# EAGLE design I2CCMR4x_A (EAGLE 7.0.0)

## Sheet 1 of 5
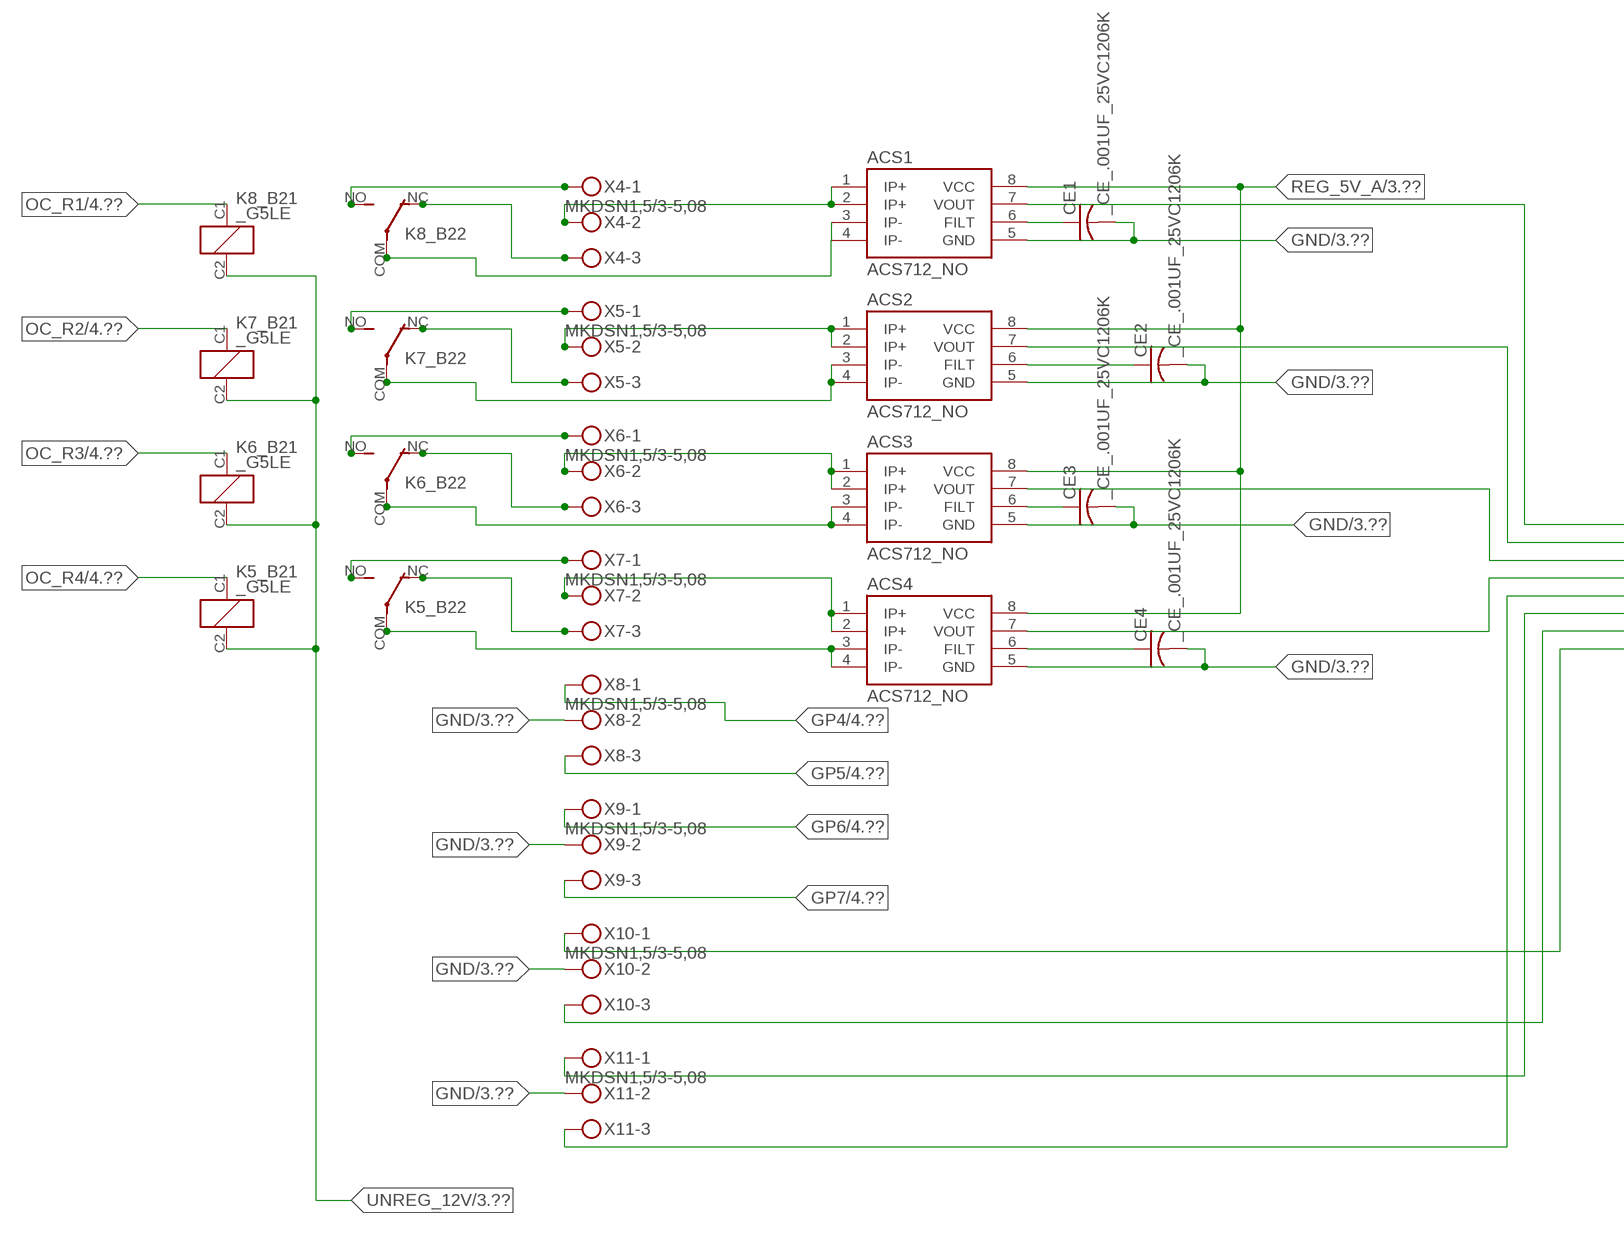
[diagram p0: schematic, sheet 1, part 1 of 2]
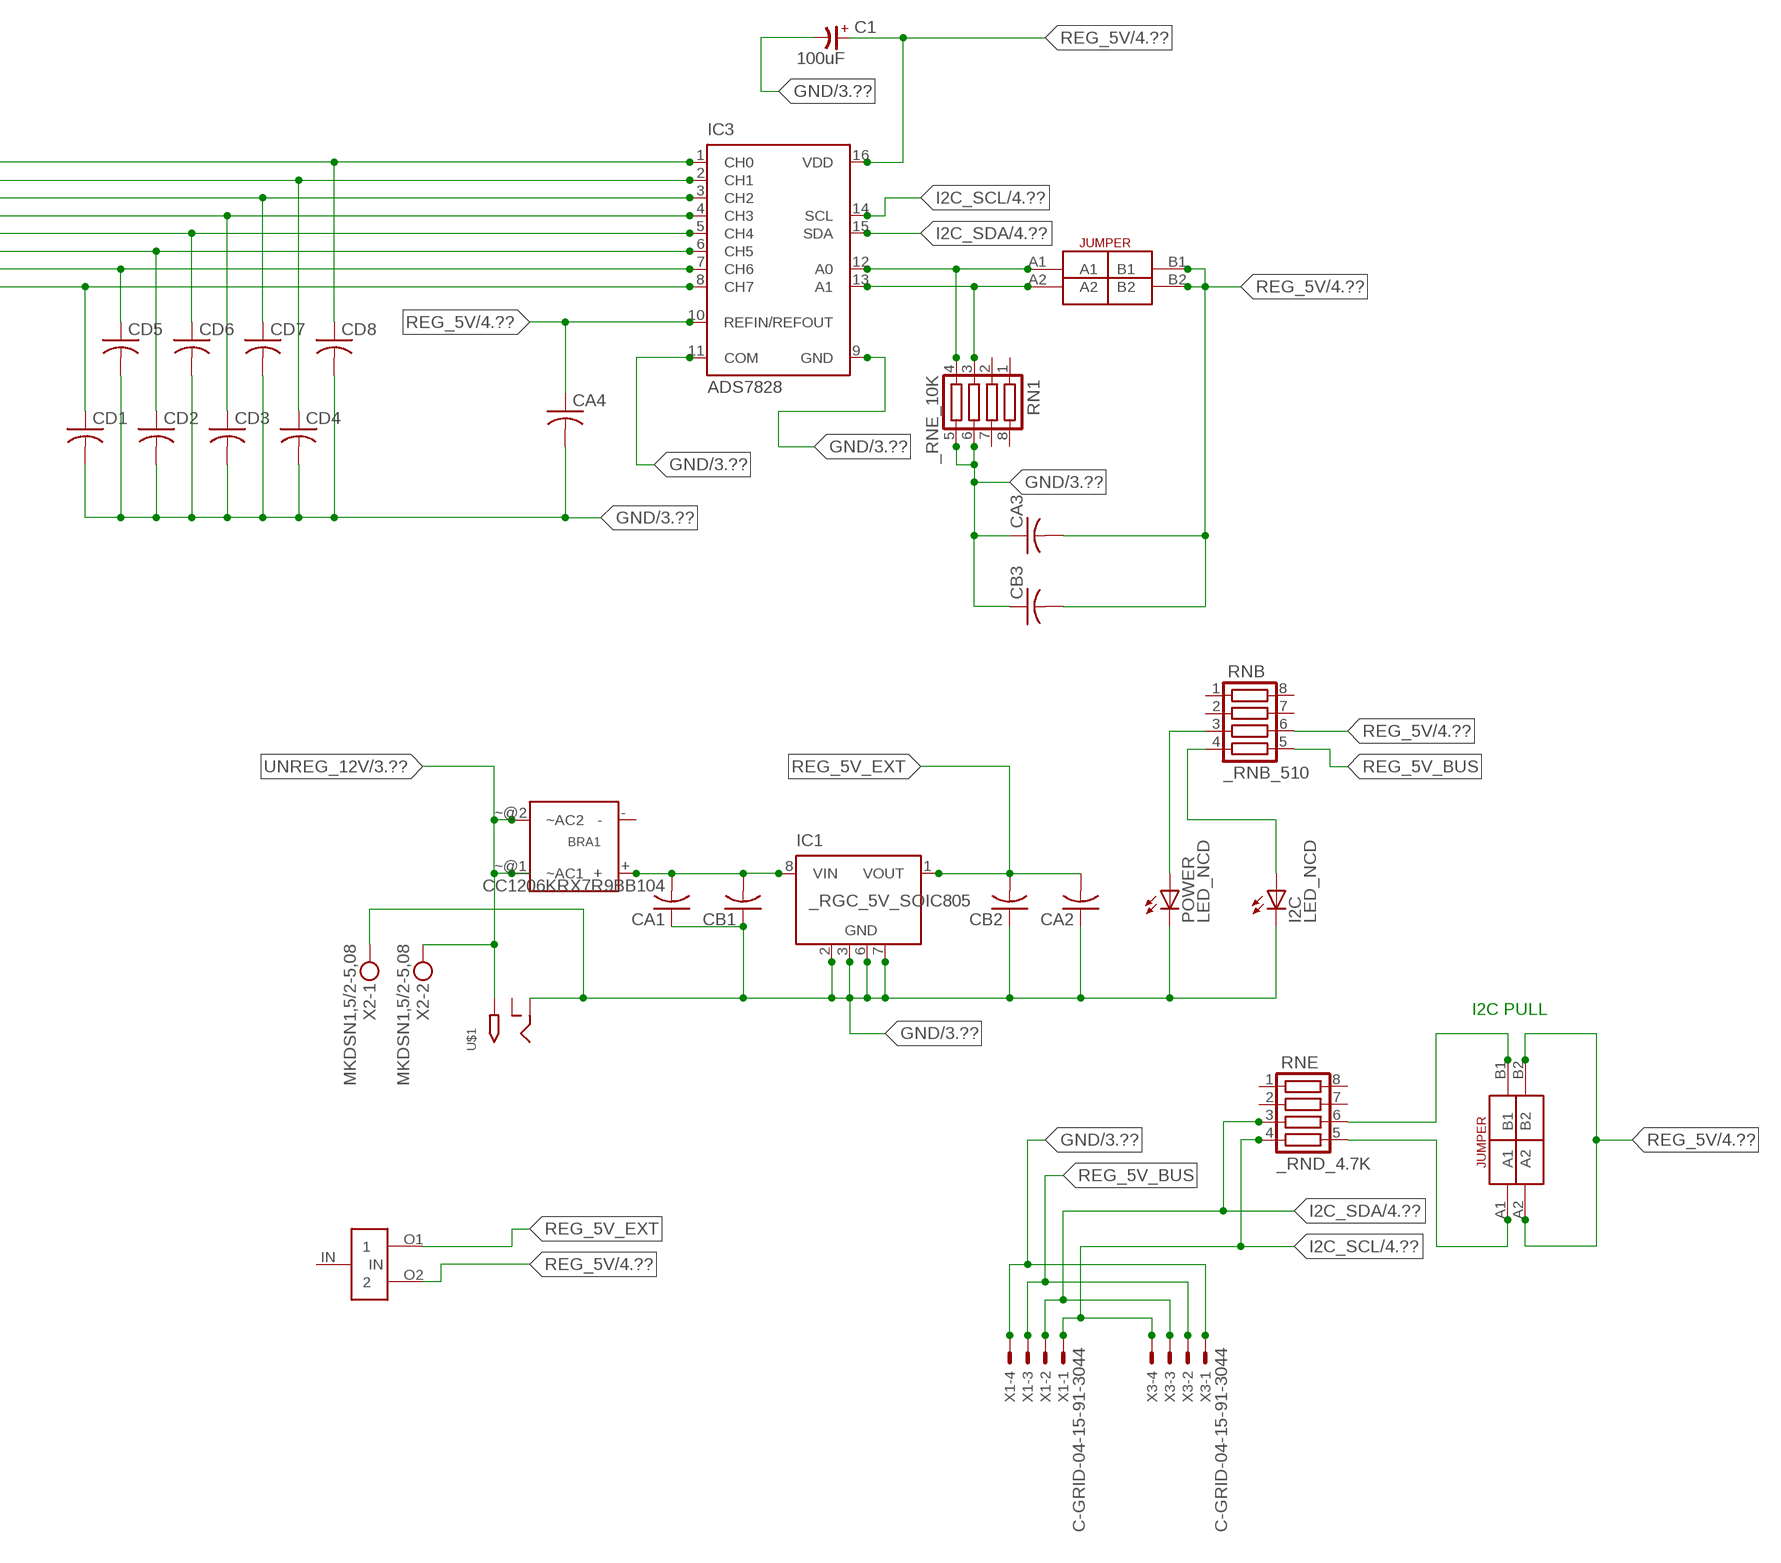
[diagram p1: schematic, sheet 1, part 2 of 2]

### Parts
ACS1  ACS712_NO  [_MA_DUAL_N-FET]
ACS2  ACS712_NO  [_MA_DUAL_N-FET]
ACS3  ACS712_NO  [_MA_DUAL_N-FET]
ACS4  ACS712_NO  [_MA_DUAL_N-FET]
BRA1  MB2S_  [MB2S]
C1  100uF  CP-E-025X060  [E-025X060]
CA1  CC1206KRX7R9BB104  [.1UF]
CA2  CC1206KRX7R9BB104C1206K  [CC1206KRX7R9BB104]
CA3  CC1206KRX7R9BB104C1206K  [CC1206KRX7R9BB104]
CA4  CC1206KRX7R9BB104C1206K  [CC1206KRX7R9BB104]
CB1  TMK316F106ZL-TC1206K  [TMK316F106ZL-T]
CB2  TMK316F106ZL-TC1206K  [TMK316F106ZL-T]
CB3  TMK316F106ZL-TC1206K  [TMK316F106ZL-T]
CD1  _CD_10NF_50VC1206K  [_CD_10NF_50V]
CD2  _CD_10NF_50VC1206K  [_CD_10NF_50V]
CD3  _CD_10NF_50VC1206K  [_CD_10NF_50V]
CD4  _CD_10NF_50VC1206K  [_CD_10NF_50V]
CD5  _CD_10NF_50VC1206K  [_CD_10NF_50V]
CD6  _CD_10NF_50VC1206K  [_CD_10NF_50V]
CD7  _CD_10NF_50VC1206K  [_CD_10NF_50V]
CD8  _CD_10NF_50VC1206K  [_CD_10NF_50V]
CE1  _CE_.001UF_25VC1206K  [CE]
CE2  _CE_.001UF_25VC1206K  [CE]
CE3  _CE_.001UF_25VC1206K  [CE]
CE4  _CE_.001UF_25VC1206K  [CE]
I2C  LED_NCD  [CHIPLED_0603]
IC1  _RGC_5V_SOIC805  [_RGC_5V_SOIC8]
IC3  ADS7828  [TSSOP16-PW]
K5_B2  _G5LE  [G5LE]
K6_B2  _G5LE  [G5LE]
K7_B2  _G5LE  [G5LE]
K8_B2  _G5LE  [G5LE]
POWER  LED_NCD  [CHIPLED_0603]
RN1  _RNE_10K  [RNE]
RNB  _RNB_510  [RNB]
RNE  _RND_4.7K  [RND]
U$1  2.1MMJACK  [PJ-102A]
U$2  LINK_2  [LINK_2]
U$3  JUMPER_2X2  [JUMPER_2X2]
U$4  JUMPER_2X2  [JUMPER_2X2]
X1  C-GRID-04-15-91-3044  [15-91-04]
X2  MKDSN1,5/2-5,08  [MKDSN1,5/2-5,08]
X3  C-GRID-04-15-91-3044  [15-91-04]
X4  MKDSN1,5/3-5,08  [MKDSN1,5/3-5,08]
X5  MKDSN1,5/3-5,08  [MKDSN1,5/3-5,08]
X6  MKDSN1,5/3-5,08  [MKDSN1,5/3-5,08]
X7  MKDSN1,5/3-5,08  [MKDSN1,5/3-5,08]
X8  MKDSN1,5/3-5,08  [MKDSN1,5/3-5,08]
X9  MKDSN1,5/3-5,08  [MKDSN1,5/3-5,08]
X10  MKDSN1,5/3-5,08  [MKDSN1,5/3-5,08]
X11  MKDSN1,5/3-5,08  [MKDSN1,5/3-5,08]

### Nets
GND: ACS1.5(GND) ACS2.5(GND) ACS3.5(GND) ACS4.5(GND) C1.- CA1.1 CA2.1 CA3.1 CA4.2 CB1.1 CB2.1 CB3.1 CD1.2 CD2.2 CD3.2 CD4.2 CD5.2 CD6.2 CD7.2 CD8.2 CE1.2 CE2.2 CE3.2 CE4.2 I2C.C IC1.2(GND) IC1.3(GND) IC1.6(GND) IC1.7(GND) IC3.9(GND) IC3.11(COM) POWER.C RN1.5 RN1.6 U$1.RING X1.4 X2.1 X3.1 X8.2 X9.2 X10.2 X11.2 ; also sheet 3,4
GP4: X8.1 ; also sheet 4
GP5: X8.3 ; also sheet 4
GP6: X9.1 ; also sheet 4
GP7: X9.3 ; also sheet 4
I2C_SCL: IC3.14(SCL) RNE.4 X1.1 X3.4 ; also sheet 4
I2C_SDA: IC3.15(SDA) RNE.3 X1.2 X3.3 ; also sheet 4
N$1: BRA1.+ CA1.2 CB1.2 IC1.8(VIN)
N$2: POWER.A RNB.3
N$3: I2C.A RNB.4
N$4: RNE.5 U$3.A1
N$5: RNE.6 U$3.B1
N$7: ACS1.1(IP+) ACS1.2(IP+) X4.2
N$8: CD5.1 IC3.7(CH6) X10.3
N$9: ACS1.7(VOUT) CD8.1 IC3.1(CH0)
N$10: ACS2.7(VOUT) CD4.1 IC3.2(CH1)
N$11: ACS3.7(VOUT) CD7.1 IC3.3(CH2)
N$12: ACS4.7(VOUT) CD3.1 IC3.4(CH3)
N$13: ACS2.1(IP+) ACS2.2(IP+) X5.2
N$17: IC3.12(A0) RN1.4 U$4.A1
N$18: IC3.13(A1) RN1.3 U$4.A2
N$20: CD2.1 IC3.6(CH5) X11.1
N$21: ACS4.1(IP+) ACS4.2(IP+) X7.2
N$22: ACS4.3(IP-) ACS4.4(IP-) K5_B2.COM(2:COM)
N$24: CD1.1 IC3.8(CH7) X10.1
N$25: CD6.1 IC3.5(CH4) X11.3
N$33: ACS1.6(FILT) CE1.1
N$34: ACS2.6(FILT) CE2.1
N$35: ACS3.6(FILT) CE3.1
N$36: ACS4.6(FILT) CE4.1
N$42: ACS1.3(IP-) ACS1.4(IP-) K8_B2.COM(2:COM)
N$43: K8_B2.NC(2:NC) X4.3
N$44: K8_B2.NO(2:NO) X4.1
N$45: K7_B2.NO(2:NO) X5.1
N$46: K6_B2.NO(2:NO) X6.1
N$137: K7_B2.NC(2:NC) X5.3
N$138: ACS2.3(IP-) ACS2.4(IP-) K7_B2.COM(2:COM)
N$139: K6_B2.NC(2:NC) X6.3
N$140: ACS3.3(IP-) ACS3.4(IP-) K6_B2.COM(2:COM)
N$141: K5_B2.NC(2:NC) X7.3
N$143: K5_B2.NO(2:NO) X7.1
N$166: ACS3.1(IP+) ACS3.2(IP+) X6.2
OC_R1: K8_B2.C1(1:C1) ; also sheet 4
OC_R2: K7_B2.C1(1:C1) ; also sheet 4
OC_R3: K6_B2.C1(1:C1) ; also sheet 4
OC_R4: K5_B2.C1(1:C1) ; also sheet 4
REG_5V: C1.+ CA3.2 CA4.1 CB3.2 IC3.10(REFIN/REFOUT) IC3.16(VDD) RNB.6 U$2.O2 U$3.A2 U$3.B2 U$4.B1 U$4.B2 ; also sheet 4
REG_5V_A: ACS1.8(VCC) ACS2.8(VCC) ACS3.8(VCC) ACS4.8(VCC) ; also sheet 3
REG_5V_BUS: RNB.5 X1.3 X3.2
REG_5V_EXT: CA2.2 CB2.2 IC1.1(VOUT) U$2.O1
UNREG_12V: BRA1.~@1(~AC1) BRA1.~@2(~AC2) K5_B2.C2(1:C2) K6_B2.C2(1:C2) K7_B2.C2(1:C2) K8_B2.C2(1:C2) U$1.TIP X2.2 ; also sheet 3,4
Unconnected: BRA1.- IC1.4(NC) IC1.5(NC) RN1.1 RN1.2 RN1.7 RN1.8 RNB.1 RNB.2 RNB.7 RNB.8 RNE.1 RNE.2 RNE.7 RNE.8 U$1.RING_SW U$2.IN

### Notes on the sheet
- I2C PULL

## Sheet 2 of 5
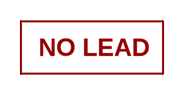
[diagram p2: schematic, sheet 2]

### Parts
U$16  NOPB_LOGO_SYM  [NOPB_LOGO_SYM]

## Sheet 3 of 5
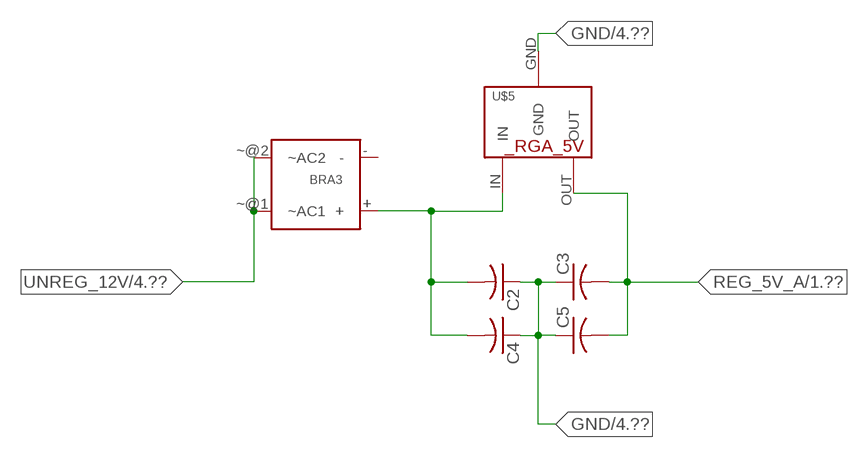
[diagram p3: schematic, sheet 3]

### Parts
BRA3  MB2S_  [MB2S]
C2  _CA_.10UF_50VC1206K  [_CA_.1UF_50V]
C3  _CA_.10UF_50VC1206K  [_CA_.1UF_50V]
C4  _CB_10UF_25VC1206K  [_CB_10UF_25V]
C5  _CB_10UF_25VC1206K  [_CB_10UF_25V]
U$5  _RGA_5V  [_RGA_5V]

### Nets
GND: C2.1 C3.1 C4.1 C5.1 U$5.GND ; also sheet 1,4
N$31: BRA3.+ C2.2 C4.2 U$5.IN
REG_5V_A: C3.2 C5.2 U$5.OUT ; also sheet 1
UNREG_12V: BRA3.~@1(~AC1) BRA3.~@2(~AC2) ; also sheet 1,4
Unconnected: BRA3.-

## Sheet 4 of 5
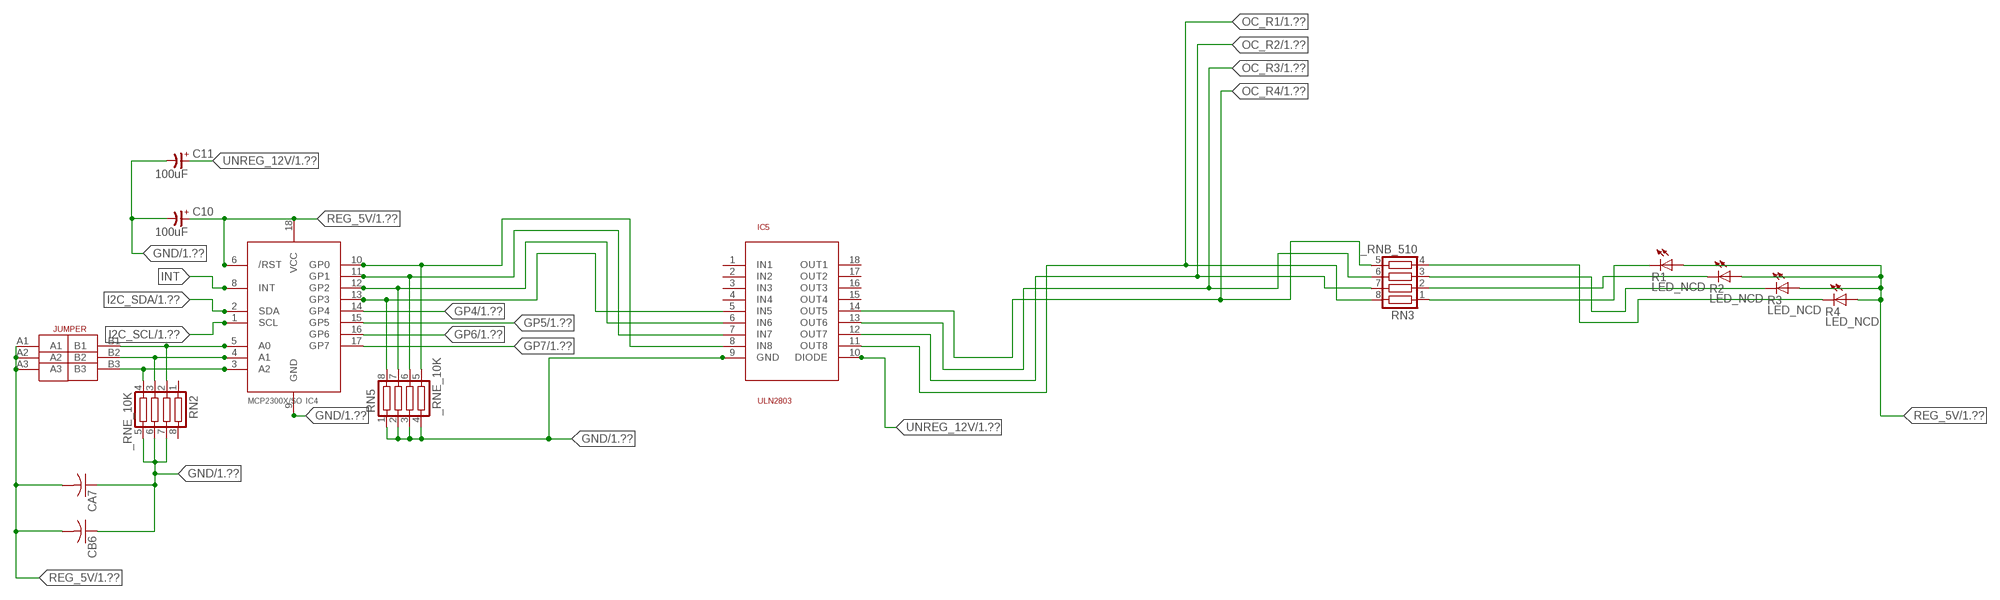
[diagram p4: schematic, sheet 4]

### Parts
C10  100uF  CP-E-025X060  [E-025X060]
C11  100uF  CP-E-025X060  [E-025X060]
CA7  CC1206KRX7R9BB104C1206K  [CC1206KRX7R9BB104]
CB6  TMK316F106ZL-TC1206K  [TMK316F106ZL-T]
IC4  MCP2300X/SO  [SO18W]
IC5  ULN2803  [SO18L]
R1  LED_NCD  [CHIPLED_0603]
R2  LED_NCD  [CHIPLED_0603]
R3  LED_NCD  [CHIPLED_0603]
R4  LED_NCD  [CHIPLED_0603]
RN2  _RNE_10K  [RNE]
RN3  _RNB_510  [RNB]
RN5  _RNE_10K  [RNE]
U$18  JUMPER_3X2  [JUMPER_3X2]

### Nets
GND: C10.- C11.- CA7.1 CB6.1 IC4.9(GND) IC5.9(GND) RN2.5 RN2.6 RN2.7 RN5.1 RN5.2 RN5.3 RN5.4 ; also sheet 1,3
GP4: IC4.14(GP4) ; also sheet 1
GP5: IC4.15(GP5) ; also sheet 1
GP6: IC4.16(GP6) ; also sheet 1
GP7: IC4.17(GP7) ; also sheet 1
I2C_SCL: IC4.1(SCL) ; also sheet 1
I2C_SDA: IC4.2(SDA) ; also sheet 1
INT: IC4.8(INT)
N$47: IC4.5(A0) RN2.2 U$18.B1
N$48: IC4.4(A1) RN2.3 U$18.B2
N$49: IC4.3(A2) RN2.4 U$18.B3
N$50: IC4.12(GP2) IC5.6(IN6) RN5.7
N$51: IC4.11(GP1) IC5.7(IN7) RN5.6
N$52: IC4.10(GP0) IC5.8(IN8) RN5.5
N$53: R1.C RN3.1
N$54: R2.C RN3.2
N$55: R3.C RN3.3
N$56: R4.C RN3.4
N$89: IC4.13(GP3) IC5.5(IN5) RN5.8
OC_R1: IC5.11(OUT8) RN3.8 ; also sheet 1
OC_R2: IC5.12(OUT7) RN3.7 ; also sheet 1
OC_R3: IC5.13(OUT6) RN3.6 ; also sheet 1
OC_R4: IC5.14(OUT5) RN3.5 ; also sheet 1
REG_5V: C10.+ CA7.2 CB6.2 IC4.6(/RST) IC4.18(VCC) R1.A R2.A R3.A R4.A U$18.A1 U$18.A2 U$18.A3 ; also sheet 1
UNREG_12V: C11.+ IC5.10(DIODE) ; also sheet 1,3
Unconnected: IC5.1(IN1) IC5.2(IN2) IC5.3(IN3) IC5.4(IN4) IC5.15(OUT4) IC5.16(OUT3) IC5.17(OUT2) IC5.18(OUT1) RN2.1 RN2.8

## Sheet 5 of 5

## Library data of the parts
ACS1-ACS4 = NCD_ULTIMATE_LIBRARY:ACS712_NO: Semiconductor Sensor Current Hall-effect-based isolated linear current sensor Digikey 620-1190-2-ND/ACS712ELCTR-20A-T
BRA1 BRA3 = NCD_ULTIMATE_LIBRARY:MB2S: Bridge Rectifier BRA MB2S 200V 500ma Digikey MB2S-TPMSTR-ND/MB2S-TP
C1 C10 C11 = NCD_ULTIMATE_LIBRARY:CP-: Capacitors All Kinds POLARIZED CAP
C2 C3 = NCD_ULTIMATE_LIBRARY:_CA_.10UF_50V: Capacitor .1uF SMT
C4 C5 = NCD_ULTIMATE_LIBRARY:_CB_10UF_25V: Capacitor 10uF SMT
CA1-CA4 CA7 = NCD_ULTIMATE_LIBRARY:CC1206KRX7R9BB104: Capacitor CA .1uF 50V SMT C1206K CC1206KRX7R9BB104
CB1-CB3 CB6 = NCD_ULTIMATE_LIBRARY:TMK316F106ZL-T: Capacitor CB 10uF SMT 1206 TMK316F106ZL-T
CD1-CD8 = NCD_ULTIMATE_LIBRARY:_CD_10NF_50V: Capacitor 10nF SMT
CE1-CE4 = NCD_ULTIMATE_LIBRARY:_CE_.001UF_25V: Capacitor .001uF SMT
I2C POWER = NCD_ULTIMATE_bhaskar:LED_NCD
IC1 = NCD_ULTIMATE_LIBRARY:_RGC_5V_SOIC8: Regulator Linear 5V Chip Positive VOLTAGE REGULATOR Digikey 497-7267-2-ND/L78L05CD13TR
IC3 = NCD_ULTIMATE_LIBRARY:ADS7828: Semiconductor ADC I2C 12-Bit, 8-Channel Sampling ANALOG-TO-DIGITAL CONVERTER Digikey 296-12402-2-ND Source: www.ti.com .. ADS7828.pdf / ADS7828E/250; MF: TEXAS INSTRUMENTS; MPN: ADS7828E/250; OC_FARNELL: 1470338; OC_NEWARK: 74C7158
IC4 = NCD_ULTIMATE_LIBRARY:MCP2300X: Semiconductor Port Expander I/O 8-Bit I2C MCP23008 Inexpensive i2c i/o expander - 8 general purpose i/o pins with optional pullups
IC5 = NCD_ULTIMATE_LIBRARY:ULN2803: Semiconductor 8 O.C. N-Channel Transistor Driver Digikey ULN2803AFWGCELTR-ND/ULN2803AFWG,C,EL
K5_B2 K6_B2 K7_B2 K8_B2 = NCD_ULTIMATE_LIBRARY:_G5LE: Relay 5A/10A SPDT; OC_FARNELL: unknown; OC_NEWARK: unknown
R1-R4 = NCD_ULTIMATE_LIBRARY:LED_NCD: LED Digikey 754-1132-2-ND/APT2012SRCPRV
RN1 RN2 RN5 = NCD_ULTIMATE_LIBRARY:_RNE_10K: Resistor Array RNE SMT 10K x 4 Single Resistor Source: http://www.ctscorp.com/components/Datasheets/CTSChipArrayDs.pdf Digikey 742C083103JPTR-ND/742C083103JP; OC_FARNELL: unknown; OC_NEWARK: unknown
RN3 RNB = NCD_ULTIMATE_LIBRARY:_RNB_510: Resistor Array RNB SMT 510 x 4 Single Resistor Source: http://www.ctscorp.com/components/Datasheets/CTSChipArrayDs.pdf Digikey 742C083511JPTR-ND/ 742C083511JP; OC_FARNELL: unknown; OC_NEWARK: unknown
RNE = NCD_ULTIMATE_LIBRARY:_RND_4.7K: Resistor Array RND SMT 4.7K x 4 Single Resistor Source: http://www.ctscorp.com/components/Datasheets/CTSChipArrayDs.pdf Digikey 742C083472JPTR-ND/742C083472JP; OC_FARNELL: unknown; OC_NEWARK: unknown
U$1 = NCD_ULTIMATE_CONNECTORS:2.1MMJACK: 2.1mm x 5.5mm DC jack with internal switch. Digikey part #PJ-102A, 4UCON part #05537 By microbuilder.eu
U$2 = NCD_ULTIMATE_LIBRARY:LINK_2: PAD_top
U$3 U$4 = NCD_ULTIMATE_CONNECTORS:JUMPER_2X2
U$5 = NCD_ULTIMATE_LIBRARY:_RGA_5V: Regulator Linear 5V Digikey 497-7255-2-ND/ L7805CDT-TR
U$16 = PatternAgents-Logos:NOPB_LOGO_SYM: NOPB_LOGO_SYM
U$18 = NCD_ULTIMATE_CONNECTORS:JUMPER_3X2
X1 X3 = NCD_ULTIMATE_CONNECTORS:C-GRID-04: CONNECTOR 4-Pos I2C wire to board 2.54 mm (0.100") pitch header Digikey WM1342-ND/0015912045; OC_FARNELL: unknown; OC_NEWARK: unknown
X2 = NCD_ULTIMATE_CONNECTORS:MKDSN1,5/2-5,08: MKDSN 1,5/ 2-5,08 Printklemme
X4-X11 = NCD_ULTIMATE_CONNECTORS:MKDSN1,5/3-5,08: MKDSN 1,5/ 3-5,08 Printklemme Nennstrom: 13,5 A Nennspannung: 250 V Rastermaß: 5,08 mm Polzahl: 3 Anschlussart: Schraubanschluss Montage: Löten Anschlussrichtung Leiter/Platine: 0 ° Artikelnummer: 1729131 Source: http://eshop.phoenixcontact.com .. 1729131.pdf

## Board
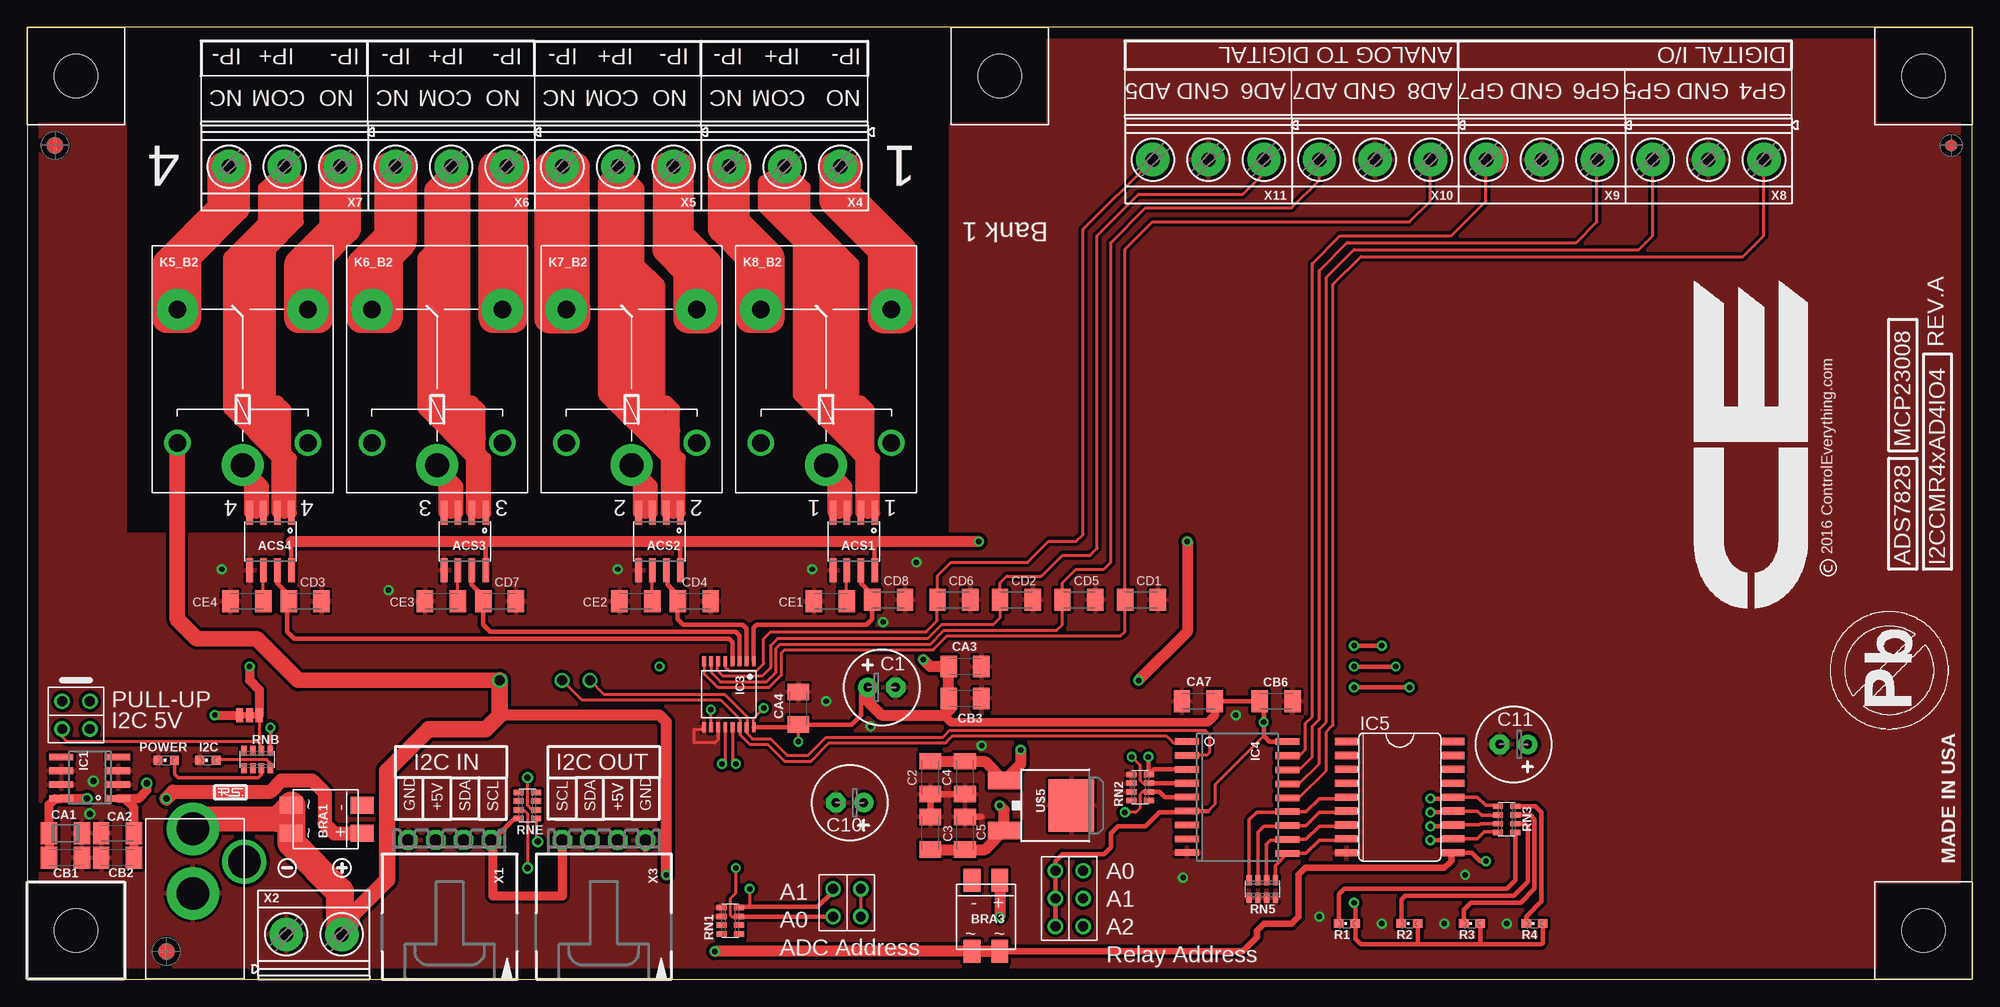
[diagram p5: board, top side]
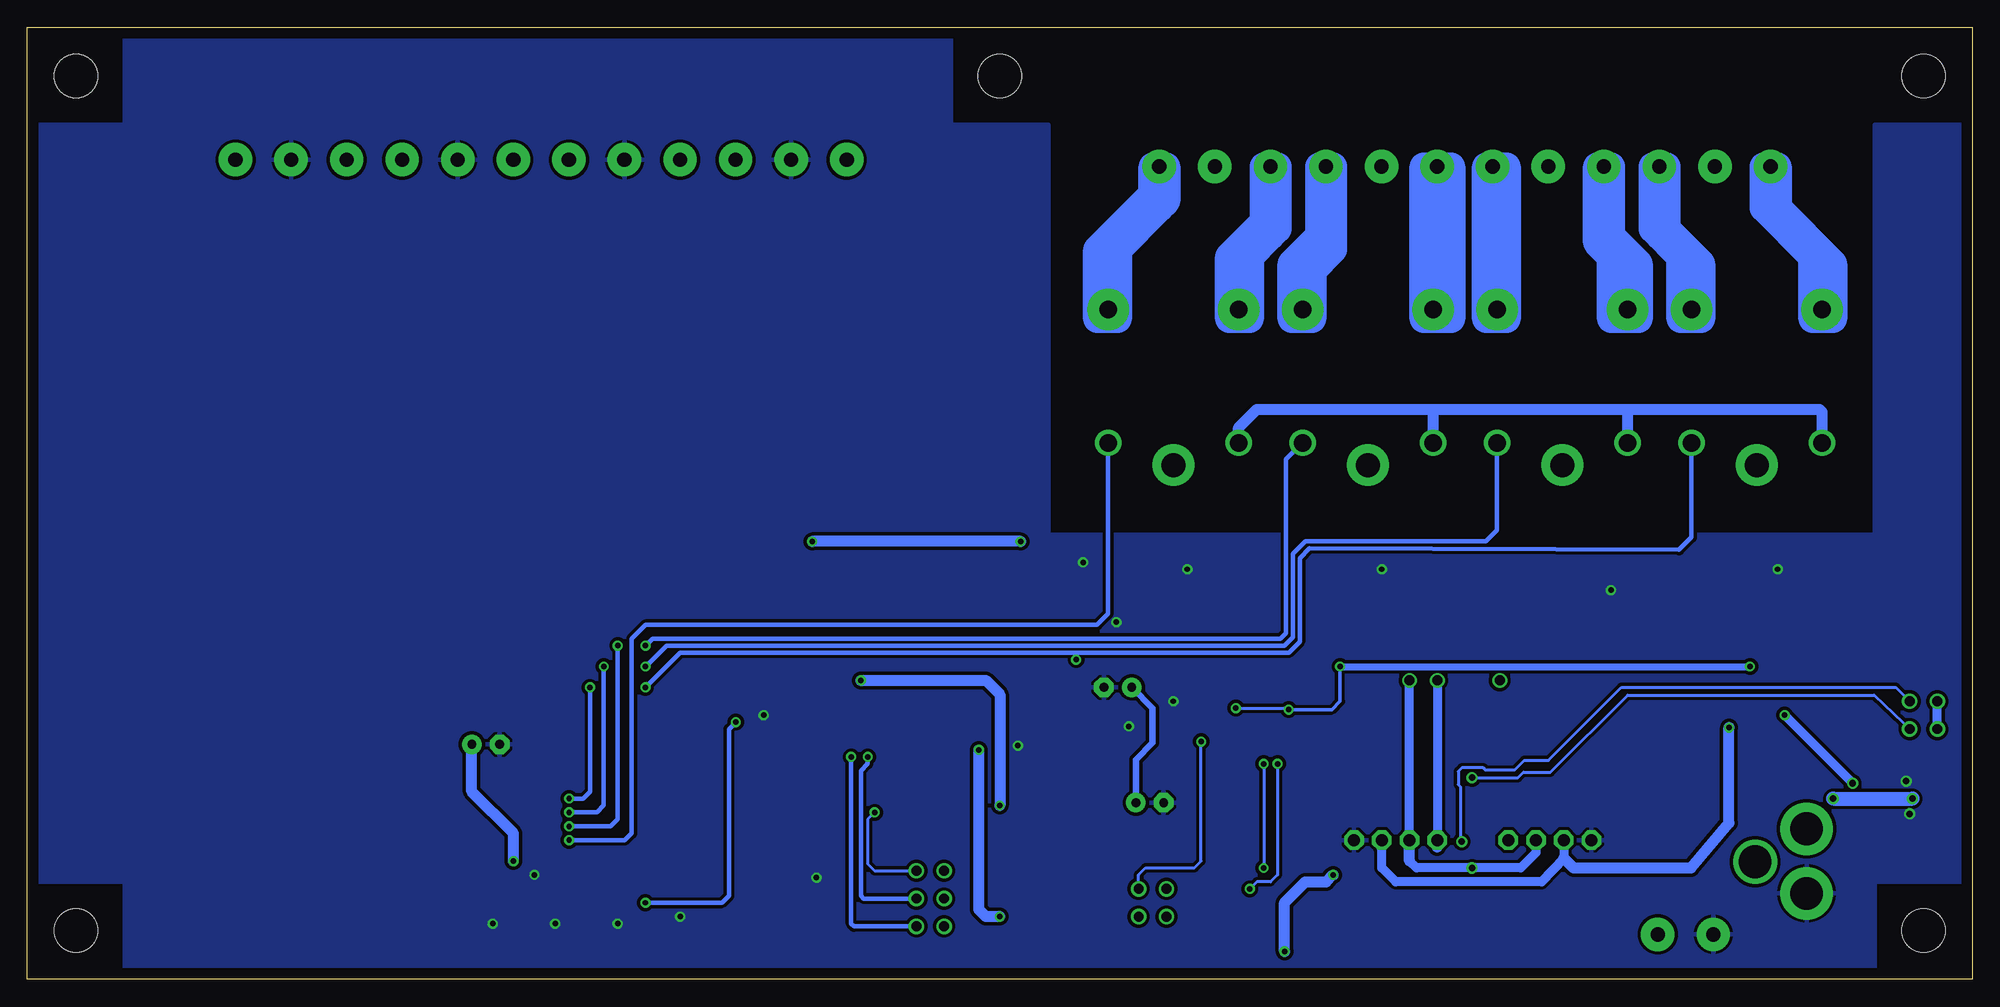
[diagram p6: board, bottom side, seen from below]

Size 177.8 x 87 mm. Coordinates in mm from the lower left corner, seen from the top.
Outline: 0,86.67 0,85.72
Outline: 0,85.72 0,0 177.8,0 177.8,87 0,87 0,85.72
Copper layers (1*16): Top 0.035mm / dielectric 1.5mm / Bottom 0.035mm
Design rules "default": minimum track width 10mil, minimum drill 24mil, track to track 8mil, track to pad 8mil, pad to pad 8mil, via to via 8mil, smd to smd 8mil, copper to edge 40mil, drill to drill 8mil, minimum pad ring 10mil, minimum via ring 8mil, stop-mask expansion 4mil, vias tented up to drill 0mil, thermal gap 10mil
Holes 3.96 mm at 4.45,4.45

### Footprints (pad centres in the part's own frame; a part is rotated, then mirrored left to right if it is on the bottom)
_MA_DUAL_N-FET = smd 0.61 x 2.21: 1 -1.905,-2.616; 2 -0.635,-2.616; 3 0.635,-2.616; 4 1.905,-2.616; 5 1.905,2.616; 6 0.635,2.616; 7 -0.635,2.616; 8 -1.905,2.616
MB2S = smd 1.55 x 2.1: + 0,-6.5; - 2.54,-6.5; ~@1 0,0; ~@2 2.54,0
E-025X060 = drill 0.813 pad 1.778: + -1.27,0 | drill 0.813 pad 1.778 octagon: - 1.27,0
_CA_.1UF_50V = smd 1.5 x 2: 1 -1.5,0; 2 1.5,0
_CB_10UF_25V = smd 1.5 x 2: 1 -1.5,0; 2 1.5,0
.1UF = smd 1.5 x 2: 1 -1.5,0; 2 1.5,0
CC1206KRX7R9BB104 = smd 1.5 x 2: 1 -1.5,0; 2 1.5,0
TMK316F106ZL-T = smd 1.5 x 2: 1 -1.5,0; 2 1.5,0
_CD_10NF_50V = smd 1.5 x 2: 1 -1.5,0; 2 1.5,0
CE = smd 1.5 x 2: 1 -1.5,0; 2 1.5,0
CHIPLED_0603 = smd 0.8 x 0.8: A 0,-0.75; C 0,0.75
_RGC_5V_SOIC8 = smd 0.6 x 2.2: 1 -1.905,-2.6; 2 -0.635,-2.6; 3 0.635,-2.6; 4 1.905,-2.6; 5 1.905,2.6; 6 0.635,2.6; 7 -0.635,2.6; 8 -1.905,2.6
TSSOP16-PW = smd 0.35 x 0.9: 1 -2.275,-3.025; 2 -1.625,-3.025; 3 -0.975,-3.025; 4 -0.325,-3.025; 5 0.325,-3.025; 6 0.975,-3.025; 7 1.625,-3.025; 8 2.275,-3.025; 9 2.275,3.025; 10 1.625,3.025; 11 0.975,3.025; 12 0.325,3.025; 13 -0.325,3.025; 14 -0.975,3.025; 15 -1.625,3.025; 16 -2.275,3.025
SO18W = smd 0.6 x 2.2: 1 -4.445,-4.6; 2 -3.175,-4.6; 3 -1.905,-4.6; 4 -0.635,-4.6; 5 0.635,-4.6; 6 1.905,-4.6; 7 3.175,-4.6; 8 4.445,-4.6; 9 5.715,-4.6; 10 5.775,4.6; 11 4.505,4.6; 12 3.235,4.6; 13 1.965,4.6; 14 0.695,4.6; 15 -0.575,4.6; 16 -1.845,4.6; 17 -3.145,4.6; 18 -4.445,4.6
SO18L = smd 0.66 x 2.032: 1 -5.08,-4.902; 2 -3.81,-4.902; 3 -2.54,-4.902; 4 -1.27,-4.902; 5 0,-4.902; 6 1.27,-4.902; 7 2.54,-4.902; 8 3.81,-4.902; 9 5.08,-4.902; 10 5.08,4.902; 11 3.81,4.902; 12 2.54,4.902; 13 1.27,4.902; 14 0,4.902; 15 -1.27,4.902; 16 -2.54,4.902; 17 -3.81,4.902; 18 -5.08,4.902
G5LE = drill 1.6: C1 -7.493,-5.969; C2 -7.493,5.969 | drill 2.2 pad 3.81: COM -9.525,0 | drill 1.6 pad 3.81: NC 4.699,5.969; NO 4.699,-5.969
CHIPLED_0603' = smd 0.8 x 0.876: A 0,-0.75; C 0,0.75
RNE = smd 0.5 x 0.9: 1 -1.2,-0.8; 2 -0.4,-0.8; 3 0.4,-0.8; 4 1.2,-0.8; 5 1.2,0.8; 6 0.4,0.8; 7 -0.4,0.8; 8 -1.2,0.8
RNB = smd 0.5 x 0.9: 1 -1.2,-0.8; 2 -0.4,-0.8; 3 0.4,-0.8; 4 1.2,-0.8; 5 1.2,0.8; 6 0.4,0.8; 7 -0.4,0.8; 8 -1.2,0.8
RND = smd 0.5 x 0.9: 1 -1.2,-0.8; 2 -0.4,-0.8; 3 0.4,-0.8; 4 1.2,-0.8; 5 1.2,0.8; 6 0.4,0.8; 7 -0.4,0.8; 8 -1.2,0.8
PJ-102A = drill 3 pad 4.8: RING 0.1,-3.39; TIP 0.1,-9.29 | drill 3 pad 3.251: RING_SW -4.6,-6.29
LINK_2 = smd 1.27 x 0.635: IN 0,0; O1 0,0.889; O2 0,-0.889
JUMPER_2X2 = drill 0.9: A1 0,2.54; A2 0,0; B1 2.54,2.54; B2 2.54,0
_RGA_5V = smd 4.826 x 4.191: GND 0,2.096 | smd 1.6 x 3: IN -2.28,-4.04; OUT 2.28,-4.04
PCB_MOUNTING_HOLE = hole 3.962: 4.445,4.445
JUMPER_3X2 = drill 0.9: A1 0,5.08; A2 0,2.54; A3 0,0; B1 2.54,5.08; B2 2.54,2.54; B3 2.54,0
15-91-04 = drill 1.1 pad 1.778 octagon: 1 -3.81,-7.62; 2 -1.27,-7.62; 3 1.27,-7.62; 4 3.81,-7.62
MKDSN1,5/2-5,08 = drill 1.3 pad 3.048: 1 -2.561,0.025; 2 2.519,0.025
MKDSN1,5/3-5,08 = drill 1.3 pad 3.048: 1 -7.641,0.025; 2 -2.561,0.025; 3 2.519,0.025

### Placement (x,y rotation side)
ACS1  75.56,40.01 180 top
ACS2  57.78,40.01 180 top
ACS3  40.01,40.01 180 top
ACS4  22.23,40.01 180 top
BRA1  24.13,13.34 90 top
BRA3  88.9,2.54 180 top
C1  78.11,26.67 0 top
C2  82.55,18.41 90 top
C3  82.55,13.34 270 top
C4  85.72,18.41 90 top
C5  85.72,13.34 270 top
C10  75.18,16.13 180 top
C11  135.89,21.46 180 top
CA1  3.49,13.34 180 top
CA2  8.26,13.34 0 top
CA3  85.72,28.57 180 top
CA4  70.48,24.77 90 top
CA7  107.06,25.4 0 top
CB1  3.49,11.11 180 top
CB2  8.26,11.11 0 top
CB3  85.72,25.65 180 top
CB6  114.17,25.4 180 top
CD1  101.85,34.67 0 top
CD2  90.42,34.67 0 top
CD3  25.4,34.54 0 top
CD4  60.96,34.54 0 top
CD5  96.14,34.67 0 top
CD6  84.71,34.67 0 top
CD7  43.18,34.54 0 top
CD8  78.74,34.67 0 top
CE1  73.41,34.54 180 top
CE2  55.63,34.54 180 top
CE3  37.85,34.54 180 top
CE4  20.07,34.54 180 top
I2C  16.51,20 90 top
IC1  5.71,18.41 90 top
IC3  64.14,26.04 180 top
IC4  110.62,17.27 270 top
IC5  125.48,16.64 270 top
K5_B2  19.68,56.52 90 top
K6_B2  37.47,56.52 90 top
K7_B2  55.24,56.52 90 top
K8_B2  73.03,56.52 90 top
POWER  12.7,20 90 top
R1  LED_NCD  [CHIPLED_0603']  120.65,5.08 90 top
R2  LED_NCD  [CHIPLED_0603']  126.36,5.08 90 top
R3  LED_NCD  [CHIPLED_0603']  132.08,5.08 90 top
R4  LED_NCD  [CHIPLED_0603']  137.79,5.08 90 top
RN1  64.26,5.33 90 top
RN2  101.73,17.53 90 top
RN3  135.25,14.61 90 top
RN5  112.9,8.26 0 top
RNB  21.02,20.07 0 top
RNE  45.72,15.88 270 top
U$1  15.24,4.45 180 top
U$2  20.32,24.13 90 top
U$3  3.17,25.4 270 top
U$4  73.66,5.71 0 top
U$5  93.34,15.88 270 top
U$10  [VISION_REF15]  12.7,2.54 0 top
U$15  PCB_MOUNTING_HOLE  [PCB_MOUNTING_HOLE]  177.8,0 90 top
U$16  176.07,22.63 90 top
U$18  93.98,4.83 0 top
U$20  PCB_MOUNTING_HOLE  [PCB_MOUNTING_HOLE]  177.8,78.11 90 top
U$21  [ICON_USA]  175.01,22.48 270 top
U$22  [ICON_MINUS]  23.75,10.16 180 top
U$23  PCB_MOUNTING_HOLE  [PCB_MOUNTING_HOLE]  93.34,78.11 90 top
U$24  [ICON_PLUS]  28.77,10.16 90 top
U$25  PCB_MOUNTING_HOLE  [PCB_MOUNTING_HOLE]  8.89,78.11 90 top
U$26  PCB_MOUNTING_HOLE  [PCB_MOUNTING_HOLE]  177.8,78.11 90 top
U$27  [VISION_REF15]  2.54,76.2 270 top
U$28  [VISION_REF10]  175.9,76.2 270 top
X1  38.61,5.08 180 top
X2  26.23,4.06 0 top
X3  52.7,5.08 180 top
X4  66.67,74.3 180 top
X5  51.44,74.3 180 top
X6  36.2,74.3 180 top
X7  20.95,74.3 180 top
X8  151.13,74.93 180 top
X9  135.89,74.93 180 top
X10  120.65,74.93 180 top
X11  105.41,74.93 180 top

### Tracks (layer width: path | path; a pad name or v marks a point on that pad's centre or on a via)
GND  (via drill 0.5, 0.6)
  Top 0.254: IC3.11 63.16,21.89 62.87,21.59 60.96,21.59 60.96,22.86 61.71,22.86 IC3.9
  Top 0.406: 34.8,12.38 X1.4
  Top 0.61: C4.1 C2.1 C3.1 | C5.1 87.22,14.84
  Top 0.813: X3.1 56.52,12.06
  other vias: 5.71,15.11 6.03,18.1 71.75,37.47 73.03,25.4 53.98,37.47 33.02,35.56 105.66,9.27 118.11,5.71 135.25,5.08 129.54,5.08 123.83,5.08 110.49,24.13 77.09,23.11 87.25,21.34 131.44,9.53 17.78,37.47 81.28,38.1 78.23,32.64
  pour Top (isolate 0.305): 8.89,-1.91 8.89,8.89 -2.54,8.89 -2.54,78.11 8.89,78.11 8.89,40.64 84.45,40.64 84.45,78.11 93.34,78.11 93.34,99.69 168.91,99.69 168.91,78.11 179.07,78.11 179.71,78.74 179.71,8.89 168.91,8.89 168.91,-1.27 168.28,-1.91
  pour Bottom (isolate 0.305): 8.89,-1.91 8.89,8.89 -10.16,8.89 -10.16,78.11 8.89,78.11 8.89,40.64 84.45,40.64 84.45,78.11 93.34,78.11 93.34,97.79 168.91,97.79 168.91,78.11 179.07,78.11 179.71,78.74 179.71,8.89 168.91,8.89 168.91,-1.27 168.28,-1.91
GP4
  Top 0.254: IC4.14 116.27,16.58 118.75,19.05 118.75,22.61 119.38,23.24 119.38,63.5 121.92,66.04 156.84,66.04 158.75,67.94 158.75,74.88 X8.1
GP5
  Top 0.254: IC4.15 116.27,17.85 118.11,19.68 118.11,22.86 118.75,23.5 118.75,64.14 121.28,66.67 147.32,66.67 148.59,67.94 148.59,74.88 X8.3
GP6
  Top 0.254: IC4.16 116.27,19.12 117.47,20.32 117.47,23.11 118.11,23.75 118.11,64.77 120.65,67.31 141.6,67.31 143.51,69.22 143.51,74.88 X9.1
GP7
  Top 0.254: IC4.17 116.3,20.42 116.84,20.95 116.84,23.37 117.47,24 117.47,65.41 120.02,67.94 130.18,67.94 133.35,71.12 133.35,74.88 X9.3
I2C_SCL  (via drill 0.9)
  Top 0.254: v48.9,27.3 50.67,25.53 63.37,25.53 65.15,23.75 65.15,23.05 | 65.15,23.05 IC3.14 | 65.15,23.05 65.15,22.35 66.04,21.46 67.69,21.46 69.22,19.94 71.63,19.94 73.28,21.59 83.95,21.59 84.58,22.23 104.14,22.23 104.78,21.59 105.89,21.59 IC4.1
  Top 0.406: RNE.4 44.51,14.68 42.55,12.7
  Top 0.813: X3.4 48.9,7.62 42.55,7.62 42.55,12.7 X1.1
  Bottom 0.813: v48.9,27.3 X3.4
  Bottom 1.016: X3.4 48.9,12.06
I2C_SDA  (via drill 0.6, 0.9)
  Top 0.254: RNE.3 45.36,15.47 45.72,15.11 v45.72,10.16 | v51.44,27.3 52.7,26.04 63.75,26.04 65.79,24 65.79,23.04 | 65.79,23.04 IC3.15 | 65.79,23.04 65.79,22.48 66.29,21.97 67.94,21.97 69.47,20.45 71.37,20.45 73.03,22.1 83.69,22.1 84.33,22.73 107.7,22.73 108.08,22.35 108.08,20.7 107.82,20.45 IC4.2
  Top 0.61: X3.3 51.44,12.06 | X1.2 39.88,12.38
  Bottom 0.813: 39.88,12.38 39.88,11.56 41.27,10.16 v45.72,10.16 50.8,10.16 51.44,10.79 | X3.3 v51.44,27.3
  Bottom 1.016: 39.88,12.38 X1.2 | 51.44,10.79 X3.3
N$1  (via drill 0.6)
  Top 0.813: CB1.2 CA1.2 1.99,15.96 2.54,16.51 IC1.8 v5.46,16.51
  Top 1.27: v12.7,16.51 13.34,17.14 22.23,17.14 23.24,18.16 26.04,18.16 27.18,17.02 27.18,14.22 28.07,13.34 BRA1.+
  Bottom 1.27: v12.7,16.51 v5.46,16.51
N$2
  Top 0.305: RNB.3 21.4,18.95 21.4,18.7 21.12,18.41 13.78,18.41 13.45,18.74 POWER.A
N$3
  Top 0.254: 22.23,18.95 22.23,19.74 21.9,20.07 16.94,20.07
  Top 0.305: RNB.4 22.23,18.95 | 16.94,20.07 I2C.A
N$4  (via drill 0.6)
  Top 0.254: RNE.5 46.52,12.6 v46.67,12.57
  Bottom 0.254: U$3.A1 6.99,26.67 32.07,26.67 38.73,20 40.96,20 41.85,19.11 44.51,19.11 44.7,19.3 46.67,19.3 46.99,18.99 46.99,17.78 46.8,17.59 46.8,12.7 v46.67,12.57
N$5  (via drill 0.6)
  Top 0.254: RNE.6 46.12,15.47 45.72,15.88 v45.72,18.41
  Bottom 0.254: v45.72,18.41 41.53,18.41 41.02,18.92 38.54,18.92 31.5,25.97 8.95,25.97 6.35,23.5 U$3.B1
N$7
  Top 1.016: ACS1.1 77.47,47.62 76.83,48.26 75.56,49.53 75.56,65.41 71.12,69.85 71.12,72.39 X4.2 67.31,72.98 67.31,70.48 70.48,67.31 70.48,53.34 76.2,47.62 ACS1.2
  Top 1.27: 76.83,48.26 76.83,52.07 76.2,52.7 76.2,49.53
  Top 1.778: 69.22,74.25 X4.2
N$8
  Top 0.254: IC3.7 62.51,28.04 63.37,27.18 67.56,27.18 68.45,28.07 68.45,30.23 68.83,30.61 82.55,30.61 83.82,31.88 94.11,31.88 94.61,32.38 94.61,34.65 CD5.1 94.64,36.22 95.89,37.47 98.42,37.47 99.06,38.1 99.06,67.31 102.23,70.48 115.57,70.48 118.11,73.03 118.11,74.88 X10.3
N$9
  Top 0.406: 77.47,34.44 CD8.1 | CD8.1 77.24,35.16 76.2,36.2 ACS1.7 | IC3.1 66.41,32.12 66.67,32.38 76.71,32.38 77.22,32.89 77.22,34.65 CD8.1
N$10
  Top 0.406: ACS2.7 58.55,37.26 58.55,36.07 59.46,35.16 CD4.1 59.44,34.52 59.44,32.89 59.94,32.38 65.41,32.38 65.76,32.03 IC3.2
N$11
  Top 0.406: ACS3.7 40.64,36.07 41.68,35.03 CD7.1 41.66,34.52 41.66,32.38 42.29,31.75 64.77,31.75 65.11,31.41 IC3.3
N$12
  Top 0.406: IC3.4 64.46,30.79 64.14,31.11 24.38,31.11 23.75,31.75 23.75,34.39 CD3.1 23.9,35.16 22.86,36.2 ACS4.7
N$13
  Top 1.016: ACS2.2 58.42,47.62 52.7,53.34 52.7,72.98 X5.2 55.24,73.02 55.25,73.02 55.88,72.39 55.88,65.41 57.78,63.5 57.78,52.7 57.78,51.44 57.78,49.53 59.05,48.26 59.69,47.62 ACS2.1
  Top 1.27: 59.05,48.26 59.05,50.16 | 59.05,50.16 57.78,51.44 57.78,50.16 58.42,49.53 | 59.05,50.16 59.05,52.07 58.42,52.7 57.78,52.7
N$17  (via drill 0.5)
  Top 0.254: IC3.12 63.81,20 v63.5,19.68 | v66.04,8.26 66.04,6.6
  Top 0.406: U$4.A1 73.66,8 72.26,6.6 66.04,6.6 65.13,6.6 RN1.4
  Bottom 0.254: v63.5,19.68 63.5,9.53 64.14,8.89 65.41,8.89 v66.04,8.26
N$18  (via drill 0.5)
  Top 0.254: IC3.13 64.46,20 v64.77,19.68 | v64.77,10.16 64.77,7.87 64.26,7.37 64.26,5.84 64.39,5.71 65.04,5.71 RN1.3
  Top 0.406: U$4.A2 65.08,5.71 RN1.3
  Bottom 0.254: v64.77,19.68 v64.77,10.16
N$20
  Top 0.254: IC3.6 63.12,29.02 63.12,28.19 63.63,27.69 67.18,27.69 67.94,28.45 67.94,30.48 68.58,31.11 82.3,31.11 83.57,32.38 88.27,32.38 88.92,33.04 CD2.1 88.92,36.22 89.53,36.83 92.71,36.83 94.61,38.73 97.16,38.73 97.79,39.37 97.79,67.94 101.6,71.75 111.12,71.75 113.03,73.66 113.03,74.88 X11.1
N$21
  Top 1.016: ACS4.2 22.86,47.62 18.41,52.07 18.41,66.04 21.59,69.22 21.59,72.34 X7.2 24.77,73.02 24.77,69.22 22.23,66.67 22.23,49.53 23.5,48.26 24.13,47.62 ACS4.1
  Top 1.27: 23.5,48.26 23.5,52.07 22.86,52.7 22.86,49.53
N$22
  Top 1.016: ACS4.4 20.32,46.35 K5_B2.COM 21.59,45.09 ACS4.3
N$23
  Top 2.54: 133.99,74.93 133.35,74.93
N$24
  Top 0.254: IC3.8 61.86,27.93 63.12,26.67 67.82,26.67 68.96,27.81 68.96,29.84 69.22,30.1 82.8,30.1 84.07,31.37 99.95,31.37 100.33,31.75 100.33,34.65 CD1.1 100.35,66.7 102.87,69.22 126.36,69.22 128.27,71.12 128.27,74.88 X10.1
N$25
  Top 0.254: IC3.5 63.81,28.52 64.14,28.19 66.67,28.19 67.31,28.83 67.31,31.11 67.94,31.75 82.17,31.75 83.19,32.77 83.19,34.65 CD6.1 83.21,36.85 84.45,38.1 91.44,38.1 93.34,40.01 95.89,40.01 96.52,40.64 96.52,68.53 X11.3 102.87,74.88 102.87,74.93
N$31  (via drill 0.5)
  Top 1.016: C2.2 C4.2 87.55,19.91 U$5.IN 90.81,19.66 v90.81,20.95 | BRA3.+ v88.9,5.71
  Bottom 1.016: v88.9,5.71 90.17,5.71 90.81,6.35 v90.81,20.95
N$33
  Top 0.254: CE1.1 74.91,37.37 ACS1.6
N$34
  Top 0.254: CE2.1 57.13,37.37 ACS2.6
N$35
  Top 0.254: CE3.1 39.35,37.37 ACS3.6
N$36
  Top 0.254: CE4.1 21.57,37.37 ACS4.6
N$42
  Top 1.016: ACS1.3 74.93,45.09 K8_B2.COM 73.66,46.35 ACS1.4
N$43
  Top 1.016: K8_B2.NC 67.06,65.66 64.14,68.58 64.14,74.25 X4.3
N$44
  Top 1.016: K8_B2.NO 78.99,66.42 74.3,71.12 74.3,74.25 X4.1
N$45
  Top 1.016: K7_B2.NO 61.21,65.15 59.05,67.31 59.05,74.25 X5.1
N$46
  Top 1.016: K6_B2.NO 43.43,73.87 X6.1
N$47  (via drill 0.5)
  Top 0.254: RN2.2 101.96,17.13 101.73,16.89 101.73,15.62 101.35,15.24 v100.33,15.24
  Top 0.406: IC4.5 104.01,16.64 103.5,17.14 102.55,17.14 RN2.2
  Bottom 0.254: v100.33,15.24 100.97,14.61 100.97,10.54 100.33,9.91 U$18.B1
N$48  (via drill 0.5)
  Top 0.254: v100.97,20.32 101.73,19.56 101.73,18.16 101.98,17.91 102.51,17.91 RN2.3
  Top 0.406: IC4.4 102.55,17.91 RN2.3
  Bottom 0.406: U$18.B2 101.35,7.37 101.6,7.62 101.6,19.05 100.97,19.68 v100.97,20.32
N$49  (via drill 0.5)
  Top 0.406: IC4.3 102.98,19.18 RN2.4 102.49,18.76 v102.49,20.32
  Bottom 0.406: U$18.B3 102.23,4.83 102.49,5.08 v102.49,20.32
N$50
  Top 0.305: RN5.7 112.5,13.44 113.03,13.97 115.15,13.97 IC4.12 116.91,14.04 118.11,15.24 120.45,15.24 IC5.6
N$51
  Top 0.305: RN5.6 113.3,12.34 113.67,12.7 115.15,12.7 IC4.11 116.91,12.77 118.11,13.97 120.45,13.97 IC5.7
N$52
  Top 0.254: 115.15,11.43 IC4.10
  Top 0.305: RN5.5 114.1,10.38 IC4.10 116.91,11.5 118.11,12.7 120.45,12.7 IC5.8
N$53
  Top 0.406: RN3.1 136.06,9.05 135.25,8.26 120.4,8.26 119.89,7.75 119.89,5.09 R1.C
N$54
  Top 0.406: RN3.2 136.93,14.21 137.16,13.97 137.16,8.89 135.89,7.62 125.98,7.62 125.6,7.24 125.6,5.09 R2.C
N$55
  Top 0.406: RN3.3 137.4,15.01 137.79,14.61 137.79,8.26 136.53,6.99 131.95,6.99 131.32,6.35 131.32,5.09 R3.C
N$56
  Top 0.406: RN3.4 137.87,15.8 138.43,15.24 138.43,7.11 137.03,5.71 137.03,5.09 R4.C
N$89
  Top 0.305: RN5.8 111.7,14.55 112.39,15.24 115.15,15.24 IC4.13 116.91,15.31 118.11,16.51 120.45,16.51 IC5.5
N$97
  Bottom 2.54: 128.27,74.88 128.29,74.91
N$103
  Bottom 2.54: 138.43,74.88 138.45,74.91
N$137
  Top 1.016: K7_B2.NC 49.28,73.91 X5.3
N$138
  Top 1.016: ACS2.4 55.88,46.35 K7_B2.COM 56.52,45.72 | ACS2.3 57.15,45.09 56.52,45.72 | 56.52,45.72 56.52,42.55
N$139
  Top 1.016: K6_B2.NC 31.5,65.79 33.66,67.94 33.66,74.25 X6.3
N$140
  Top 1.016: ACS3.4 38.1,46.35 K6_B2.COM 39.37,45.09 ACS3.3
N$141
  Top 1.016: K5_B2.NC 13.72,66.42 18.41,71.12 18.41,74.25 X7.3
N$143
  Top 1.016: K5_B2.NO 25.65,65.66 28.57,68.58 28.57,74.25 X7.1
N$162
  Top 1.016: 20.95,45.09 20.95,42.55
N$163
  Top 1.016: 23.5,47.62 23.5,42.55
N$164
  Top 1.016: 21.59,49.53 21.59,67.31 24.13,69.85 24.13,72.39 23.5,73.03 22.86,72.39 | 22.86,72.39 22.23,71.75 22.23,69.22 23.5,70.48 23.5,71.75 22.86,72.39 | 22.86,72.39 22.86,69.22 19.05,65.41 19.05,52.7 20.95,50.8 20.95,51.44 20.95,66.04 | 20.95,66.67 20.95,66.04 | 20.95,66.04 19.68,64.77 19.68,53.34 20.32,52.7 20.32,64.77
  Top 1.27: 20.95,50.16 20.95,51.44
N$165
  Top 1.016: 38.73,45.09 38.73,42.55
N$166
  Top 1.016: 41.27,47.62 41.27,42.55 | ACS3.2 40.64,47.62 36.2,52.07 36.2,66.04 36.83,66.67 36.83,72.34 X6.2 40.01,73.02 40.01,50.8 40.01,49.53 41.91,47.62 ACS3.1
  Top 1.27: 41.27,47.62 41.27,49.53 | 41.27,49.53 40.01,50.8 | 39.37,50.16 40.01,49.53 | 41.27,49.53 41.27,52.07 40.64,52.7 40.64,50.8
N$167
  Top 1.016: 39.37,49.53 37.47,51.44 | 37.47,51.44 36.83,52.07 36.83,65.41 38.1,66.67 38.1,73.66 38.73,74.3 38.73,66.04 | 38.73,66.04 38.73,51.44 39.37,50.8 39.37,73.03 | 37.47,72.39 37.47,51.44 | 37.47,51.44 38.1,52.07 38.1,65.41 38.73,66.04
N$168
  Top 1.016: 59.05,47.62 59.05,42.55
N$170
  Top 1.016: 56.52,63.5 55.88,63.5 53.98,65.41 53.98,72.39 54.61,72.39 | 57.15,49.53 53.34,53.34 53.34,72.39 53.98,73.03 54.61,72.39 | 54.61,72.39 55.24,71.75 55.24,52.07 55.88,51.44 | 55.88,51.44 57.15,50.16 57.15,63.5 55.88,64.77 55.88,51.44 | 55.88,51.44 56.52,52.07 56.52,62.87 | 54.61,72.39 54.61,53.34 | 54.61,52.7 54.61,53.34 | 54.61,53.34 53.98,53.98 53.98,64.77
N$171
  Top 1.016: 74.3,45.09 74.3,42.55
N$172
  Top 1.016: 76.83,47.62 76.83,42.55
N$173
  Top 1.016: 70.48,69.85 70.48,72.39 69.22,73.66 68.58,73.03 67.94,73.03 67.94,71.12 71.12,67.94 71.12,53.34 74.93,49.53 74.93,50.16 | 70.48,69.85 70.48,69.22 74.93,64.77 74.93,50.8 | 70.48,69.85 68.58,71.75 68.58,72.39 69.22,73.03 69.85,72.39 69.85,71.75 | 69.85,71.12 69.85,71.75 | 69.85,71.75 69.22,72.39
N$174
  Top 1.016: 74.3,50.8 74.3,64.77 71.75,67.31 71.75,53.34 72.39,52.7 | 73.03,52.07 73.66,51.44 73.66,64.77 72.39,66.04 72.39,52.7 | 72.39,52.7 73.03,52.07 | 73.03,52.07 73.03,64.77
N$305
  Top 2.54: 64.16,74.27 64.16,68.56 66.67,66.04 66.67,61.59 67.06,61.21
N$306
  Top 2.54: 74.32,74.27 74.32,71.1 78.74,66.67 78.74,61.47 78.99,61.21
N$307
  Top 2.54: 59.08,74.27 59.08,67.29 60.96,65.41 60.96,61.47 61.21,61.21
N$308
  Top 2.54: 43.84,74.27 43.84,61.62 43.43,61.21
N$309
  Top 2.54: 48.92,74.27 48.92,61.57 49.28,61.21
N$311
  Top 2.54: 33.68,74.27 33.68,67.33 31.75,65.41 31.75,61.47 31.5,61.21
N$313
  Top 2.54: 18.44,74.27 18.44,70.51 13.34,65.41 13.34,61.59 13.72,61.21
N$315
  Top 2.54: 28.6,74.27 28.6,68.6 25.4,65.41 25.4,61.47 25.65,61.21
N$360
  Top 2.54: 28.6,74.27 28.6,68.6 26.04,66.04 26.04,61.59 25.65,61.21
N$361
  Top 2.54: 18.44,74.27 18.44,70.51 13.97,66.04 13.97,61.47 13.72,61.21
N$363
  Top 2.54: 43.84,74.27 43.84,61.62 43.43,61.21
N$364
  Top 2.54: 33.68,74.27 33.68,67.33 31.75,65.41 31.75,61.47 31.5,61.21
N$366
  Top 2.54: 59.08,74.27 59.08,66.65 60.96,64.77 60.96,61.47 61.21,61.21
N$367
  Top 2.54: 48.92,74.27 48.92,61.57 49.28,61.21
N$369
  Top 2.54: 74.32,74.27 74.32,71.1 78.74,66.67 78.74,61.47 78.99,61.21
N$370
  Top 2.54: 64.16,74.27 64.16,69.19 67.31,66.04 67.31,61.47 67.06,61.21
N$373
  Bottom 2.54: 13.72,61.21 13.72,65.79 18.41,70.48 18.41,74.25 18.44,74.27
N$374
  Bottom 2.54: 25.65,61.21 25.65,65.02 28.57,67.94 28.57,74.25 28.6,74.27
N$375
  Bottom 2.54: 43.43,61.21 43.43,63.75 43.81,64.14 43.81,74.25 43.84,74.27
N$376
  Bottom 2.54: 61.21,61.21 61.21,64.52 59.05,66.67 59.05,74.25 59.08,74.27
N$377
  Bottom 2.54: 31.5,61.21 31.5,64.52 33.66,66.67 33.66,74.25 33.68,74.27
N$379
  Bottom 2.54: 49.28,61.21 49.28,63.75 48.9,64.14 48.9,72.98 48.92,74.27
N$380
  Top 2.54: 48.9,63.5 48.9,74.3 49.53,74.3 49.53,63.5 | 48.9,63.5 49.53,63.5 | 49.53,63.5 49.53,62.87 | 49.53,62.87 49.53,60.96 48.9,60.96 48.9,61.59 | 48.9,61.59 48.9,62.87 | 48.9,63.5 48.9,62.87 | 48.9,62.87 49.53,62.87 | 48.9,61.59 50.16,61.59 | 50.16,61.59 50.16,74.3 47.62,74.3 47.62,60.33 50.16,60.33 50.16,61.59
N$383
  Top 2.54: 58.42,74.3 58.42,66.67 60.33,64.77 60.33,60.33 62.23,60.33 62.23,65.41 59.69,67.94 59.69,74.3 58.42,74.3
N$384
  Top 2.54: 66.04,60.33 66.04,66.04 63.5,68.58 63.5,74.3 64.77,74.3 64.77,69.22 67.94,66.04 67.94,60.33 66.04,60.33
N$386
  Top 2.54: 73.66,74.3 73.66,71.12 78.11,66.67 78.11,60.33 80.01,60.33 80.01,66.67 74.93,71.75 74.93,74.3 73.66,74.3
N$387
  Top 2.54: 44.45,74.3 44.45,60.33 42.55,60.33 42.55,74.3 44.45,74.3
N$389
  Top 2.54: 34.29,74.3 34.29,67.31 33.02,66.04 33.02,60.33 30.48,60.33 30.48,65.41 33.02,67.94 33.02,74.3 34.29,74.3
N$390
  Top 2.54: 28.57,74.3 29.21,74.3 29.21,68.58 26.67,66.04 26.67,60.33 24.77,60.33 24.77,65.41 27.94,68.58 | 28.57,69.22 28.57,74.3 | 28.57,74.3 27.94,74.3 27.94,67.94
N$392
  Top 2.54: 19.05,74.3 19.05,70.48 14.61,66.04 14.61,60.33 12.7,60.33 12.7,65.41 17.78,70.48 17.78,74.3 19.05,74.3
N$393
  Bottom 2.54: 18.41,74.3 17.78,74.3 17.78,70.48 12.7,65.41 12.7,60.33 14.61,60.33 14.61,66.04 19.05,70.48 19.05,74.3
N$395
  Bottom 2.54: 27.94,74.3 27.94,68.58 24.77,65.41 24.77,60.33 26.67,60.33 26.67,66.04 29.21,68.58 29.21,74.3 27.94,74.3
N$396
  Bottom 2.54: 33.02,74.3 33.02,67.94 30.48,65.41 30.48,60.33 33.02,60.33 33.02,66.04 34.29,67.31 34.29,74.3 33.02,74.3
N$398
  Bottom 2.54: 44.45,74.3 42.55,74.3 42.55,60.33 44.45,60.33 44.45,74.3
N$399
  Bottom 2.54: 47.62,74.3 47.62,60.33 50.16,60.33 50.16,74.3 47.62,74.3
N$401
  Bottom 2.54: 58.42,74.3 58.42,66.67 60.33,64.77 60.33,60.33 62.23,60.33 62.23,65.41 59.69,67.94 59.69,74.3 58.42,74.3
N$402
  Bottom 2.54: 67.06,61.21 67.06,65.02 66.04,66.04 | 66.04,66.04 64.14,67.94 | 64.14,67.94 64.14,74.25 64.16,74.27 | 64.14,67.94 63.5,68.58 63.5,74.3 64.77,74.3 64.77,69.22 67.94,66.04 67.94,60.33 66.04,60.33 66.04,66.04
N$404
  Bottom 2.54: 78.99,61.21 78.99,65.79 78.11,66.67 | 78.11,66.67 74.3,70.48 | 74.3,70.48 74.3,74.25 74.32,74.27 | 74.3,70.48 73.66,71.12 73.66,74.3 74.93,74.3 74.93,71.75 80.01,66.67 80.01,60.33 78.11,60.33 78.11,66.67
OC_R1  (via drill 0.5)
  Top 0.305: IC5.11 132.59,12.83 133.22,13.46 134.4,13.46 RN3.8
  Top 0.406: v128.27,12.7 130.25,12.7 IC5.11
  Bottom 0.406: K8_B2.C1 78.99,33.4 80.01,32.38 121.28,32.38 122.56,31.11 122.56,13.34 123.19,12.7 v128.27,12.7
OC_R2  (via drill 0.5)
  Top 0.305: IC5.12 132.72,14.1 132.84,14.22 134.44,14.22 RN3.7
  Top 0.406: v128.27,13.97 130.25,13.97 IC5.12 | v121.28,30.48 v123.83,30.48
  Bottom 0.406: K7_B2.C1 62.74,47.5 62.74,31.62 63.25,31.11 120.65,31.11 v121.28,30.48 | v123.83,30.48 123.83,14.61 124.46,13.97 v128.27,13.97
OC_R3  (via drill 0.5)
  Top 0.305: IC5.13 132.59,15.37 132.97,14.99 134.44,14.99 RN3.6
  Top 0.406: v128.27,15.24 130.25,15.24 IC5.13 | v121.28,28.57 v125.09,28.57
  Bottom 0.406: 128.4,15.37 v128.27,15.24 125.73,15.24 125.09,15.88 v125.09,28.57 | K6_B2.C1 43.43,41.02 44.45,40.01 60.96,40.01 62.1,38.86 62.1,31.24 62.87,30.48 119.38,30.48 v121.28,28.57
OC_R4  (via drill 0.5)
  Top 0.305: IC5.14 132.59,16.64 133.35,15.88 134.38,15.88 RN3.5
  Top 0.406: v128.27,16.51 130.25,16.51 IC5.14 | v121.28,26.67 v126.36,26.67
  Bottom 0.406: 128.4,16.64 v128.27,16.51 127,16.51 126.36,17.14 v126.36,26.67 | K5_B2.C1 25.65,40.39 26.8,39.24 60.58,39.37 61.47,38.48 61.47,30.86 62.48,29.84 118.11,29.84 v121.28,26.67
REG_5V  (via drill 0.5)
  Top 0.254: RNB.6 21.42,21.29 21.21,21.5 | 21.21,21.5 20.99,21.72 3.62,21.72 3.17,22.16 U$3.B2 | U$4.B2 U$4.B1 | v70.48,21.72 CA4.1 | U$2.O2 21.21,21.5 | 113.03,22.23 108.58,17.78 108.58,16 107.95,15.37 | IC3.16 66.41,23.86 v67.31,24.77 | v62.48,24.64 62.48,23.04 IC3.10
  Top 0.406: IC3.16 70.23,23.01 CA4.1 75.33,23.27 76.2,24.13 76.2,26.04 C1.+ | CB3.2 84.22,25.17 | IC4.18 113.54,21.72 113.03,22.23 v113.03,23.5 113.03,25.68 CB6.2 CA7.2 | 127,3.17 121.92,3.17 121.4,3.69 R1.A 121.4,6.87 v121.28,6.99 | 127,3.17 132.72,3.17 | 132.72,3.17 138.43,3.17 138.54,3.29 R4.A | R3.A 132.83,3.29 132.72,3.17 | R2.A 127.11,3.29 127,3.17 | 107.95,15.37 IC4.6 105.89,15.24 103.5,15.24 102.23,13.97 99.69,13.97 99.06,13.34 99.06,12.06 98.42,11.43 94.61,11.43 93.98,10.79 U$18.A1 U$18.A2 U$18.A3
  Top 0.762: 83.82,24.13 84.45,23.5 107.95,23.5 108.58,24.13 108.58,25.38
  Top 0.813: v20.32,28.57 20.32,27.3 21.21,26.42 U$2.O2
  Top 1.016: C1.+ 76.83,25.4 78.11,24.13 83.82,24.13 84.45,24.77 84.45,25.42 CB3.2 CA3.2 82.55,28.57 v81.92,29.21 | 108.58,25.38 CA7.2
  Bottom 0.254: U$4.B1 76.2,9.53 75.56,10.16 71.12,10.16 70.48,10.79 v70.48,21.72 | v67.31,24.77 62.87,24.77 v62.48,24.64
  Bottom 0.305: v62.48,24.64 58.55,24.64 57.78,25.4 v57.78,28.57
  Bottom 0.406: v121.28,6.99 114.3,6.99 113.67,7.62 113.67,22.86 v113.03,23.5
  Bottom 0.61: C10.+ 76.45,20.07 74.93,21.59 74.93,24.77 C1.+
  Bottom 0.635: v57.78,28.57 v20.32,28.57
  Bottom 0.813: U$3.B2 U$3.A2
REG_5V_A  (via drill 0.5)
  Top 0.406: ACS1.8 77.47,40.01 | ACS2.8 59.69,40.01 | ACS3.8 41.91,40.01 | ACS4.8 24.13,40.01
  Top 1.016: C3.2 C5.2 87.55,11.84 U$5.OUT 89.31,15.47 v88.9,15.88 | 24.13,40.01 41.91,40.01 59.69,40.01 77.47,40.01 v87,40.01 | v106.05,40.01 106.05,31.75 v101.6,27.3
  Bottom 1.016: v87,40.01 v106.05,40.01 | v101.6,27.3 90.17,27.3 88.9,26.04 v88.9,15.88
REG_5V_BUS  (via drill 0.5)
  Top 0.305: RNB.5 22.26,22.9 v22.23,22.99
  Top 0.61: X1.3 37.34,12.38 | X3.2 53.98,12.06
  Bottom 0.813: 37.34,12.38 37.34,11.05 39.37,8.89 52.7,8.89 53.98,10.16 53.98,12.06
  Bottom 1.016: v22.23,22.99 22.23,14.29 25.72,10.16 36.45,10.16 37.34,11.05 | 37.34,12.38 X1.3 | 53.98,12.06 X3.2
REG_5V_EXT  (via drill 0.5, 0.6)
  Top 0.813: CB2.2 CA2.2 9.76,15.64 8.89,16.51 | 8.89,16.51 IC1.1 | v10.92,17.91 10.92,17.27 10.16,16.51 8.89,16.51 | v17.14,24.13 U$2.O1
  Bottom 0.813: v17.14,24.13 v10.92,17.91
UNREG_12V  (via drill 0.5, 0.9)
  Top 0.406: v133.35,10.79 132.84,10.79 132.08,11.56 IC5.10
  Top 0.61: BRA3.~@1 111.12,2.54 112.39,3.81 112.39,4.45 113.03,5.08 115.57,5.08 116.2,5.71 116.2,9.53 116.84,10.16 129.54,10.16 130.18,10.79 130.18,11.35 IC5.10
  Top 1.016: BRA3.~@2 BRA3.~@1 v62.87,2.54 | v58.42,9.53 58.42,23.5 57.78,24.13 43.81,24.13 43.18,24.77
  Top 1.422: v43.18,27.3 24.77,27.3 20.95,31.11 15.49,31.11 13.72,32.89 K5_B2.C2
  Top 1.524: v43.18,27.3 43.18,24.77 43.18,24.13 41.91,22.86 36.7,22.86 32.89,19.05 32.89,9.08 29.11,5.3 28.57,4.76
  Top 2.286: BRA1.~@2 22.86,14.61 16.01,14.61
  Top 2.54: 16.01,14.61 U$1.TIP | X2.2 28.55,4.45 28.57,4.76 | BRA1.~@2 BRA1.~@1 24.13,12.45 28.57,8 28.57,5.84 29.11,5.3
  Bottom 1.016: v62.87,2.54 62.87,6.99 60.96,8.89 59.05,8.89 v58.42,9.53 | 67.31,48.77 K8_B2.C2 67.06,50.42 65.41,52.07 49.53,52.07 | 49.53,52.07 31.75,52.07 | 31.75,52.07 13.97,52.07 13.72,51.82 K5_B2.C2 | K6_B2.C2 31.5,51.82 31.75,52.07 | K7_B2.C2 49.28,51.82 49.53,52.07 | v133.35,10.79 133.35,13.34 137.16,17.14 C11.+

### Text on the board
tNames: IP- | IP+ | IP- | IP- | IP+ | IP- | IP- | IP+ | IP- | IP- | IP+ | IP- | ANALOG TO DIGITAL | DIGITAL I/O | AD5 | GND | AD6 | AD7 | GND | AD8 | GP7 | GND | GP6 | GP5 | GND | GP4 | NC | COM | NO | NC | COM | NO | NC | COM | NO | NC | COM | NO | 4 | 1 | Bank 1 | REV.A | MCP23008 | 4 | 4 | 3 | 3 | 2 | 2 | 1 | 1 | 2016 ControlEverything.com | ADS7828 | I2CCMR4xAD4IO4 | PULL-UP | I2C 5V | I2C IN | I2C OUT | GND | +5V | SDA | SCL | SCL | SDA | +5V | +5V | GND | A0 | A1 | A1 | A0 | A2 | ADC Address | Relay Address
